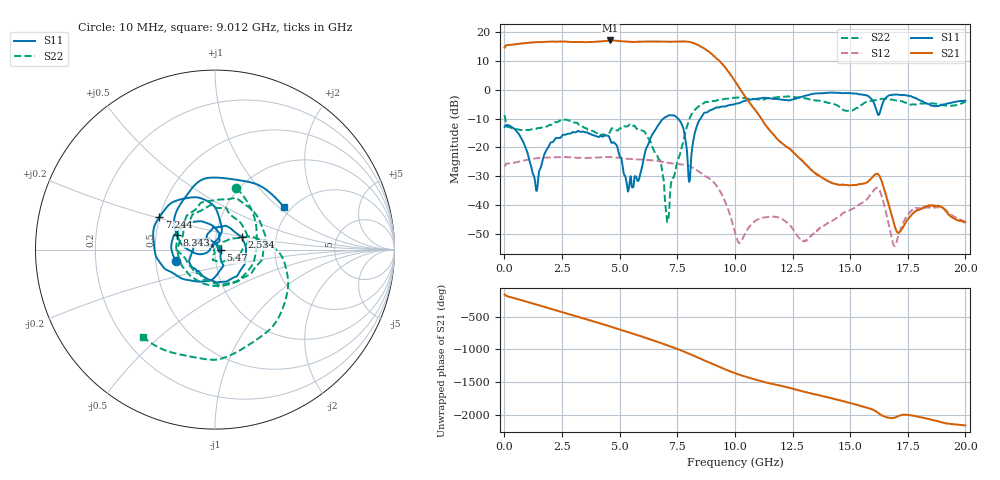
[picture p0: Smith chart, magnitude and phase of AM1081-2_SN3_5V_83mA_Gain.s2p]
!Agilent Technologies,E8364B,MY43040894,A.07.50.67
!Agilent E8364B: A.07.50.67
!Date: Wednesday, June 23, 2021 08:06:43
!Correction: S11(Full 2 Port(1,2))
!S21(Full 2 Port(1,2))
!S12(Full 2 Port(1,2))
!S22(Full 2 Port(1,2))
!S2P File: Measurements: S11, S21, S12, S22:
# Hz S  dB  R 50
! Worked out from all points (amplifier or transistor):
!   3201 points, 10 MHz to 20 GHz, reference 50 ohm
!   highest |S21| = 17.0 dB at 4.601 GHz (marker M1)
!   |S21| within 3 dB of that: start of sweep to 8.712 GHz
!   unconditionally stable (mu >= 1): start of sweep to end of sweep
!   at 3.34 GHz: K = 1.20, MAG = 17.3 dB, |S12| = -23.6 dB
!   at 10.01 GHz: K = 33.90, MAG = 7.8 dB, |S12| = -49.3 dB
!   at 20 GHz: K = 6904.74, MAG = -41.5 dB, |S12| = -45.6 dB
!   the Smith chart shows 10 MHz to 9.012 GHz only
!   S11 on the Smith chart (normalised r, x): 10 MHz: 0.64, -0.09; 2.534 GHz: 1.34, +0.19; 5.47 GHz: 1.06, -0.00; 7.244 GHz: 0.50, +0.21; 8.343 GHz: 0.64, +0.11; 9.012 GHz: 1.83, +1.09
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1e7  -12.89 -163.6  14.55 -163.7  -26.65 15.6  -8.82 70.8
5.972062e8  -15.05 116.6  15.83 124.3  -24.97 -44.8  -13.76 -83.3
1.078216e9  -24.22 65.2  16.20 75.6  -24.15 -86.8  -13.96 -144.8
1.821594e9  -20.99 120.8  16.55 -1.2  -23.49 -157.2  -12.80 141.8
2.533738e9  -15.61 25.2  16.63 -75.5  -23.32 134.5  -10.28 63.2
3.345831e9  -14.52 -66.4  16.50 -159.8  -23.59 55.5  -12.41 -34.4
3.895556e9  -15.83 -115.2  16.54 143.7  -23.52 3.3  -14.57 -91.6
4.601453e9  -17.61 -170.4  17.01 67.3  -23.31 -68.5  -14.27 -173.7
5.038734e9  -23.36 115.8  16.78 17.3  -23.67 -114.0  -13.35 142.4
5.469769e9  -30.09 -3.1  16.50 -30.1  -24.03 -157.6  -12.11 94.0
6.075716e9  -22.77 -61.8  16.60 -98.1  -24.27 138.5  -14.55 13.1
6.675416e9  -12.26 -138.2  16.61 -169.8  -24.73 70.8  -23.93 -84.1
7.243881e9  -8.90 149.7  16.58 120.1  -25.48 4.2  -31.68 39.6
7.587459e9  -10.47 106.2  16.65 75.0  -25.78 -37.9  -23.14 40.8
7.918544e9  -21.12 69.5  16.58 27.7  -26.11 -82.9  -12.80 17.4
8.343331e9  -12.81 158.5  15.68 -37.6  -27.83 -143.8  -6.37 -34.9
9.011747e9  -6.92 31.6  12.22 -139.5  -31.52 123.6  -4.00 -129.4
9.50525e9  -5.85 -66.2  8.33 146.0  -37.49 44.6  -3.25 146.4
1.0005e10  -4.92 -164.4  2.95 75.8  -49.28 -50.4  -2.83 69.3
1.334083e10  -1.55 176.1  -27.94 123.9  -50.35 87.2  -3.57 3.7
1.667042e10  -2.05 13.5  -39.76 116.0  -46.42 113.1  -3.26 -80.6
2e10  -3.83 112.8  -45.87 -1.8  -45.58 -3.9  -4.34 -131.7
